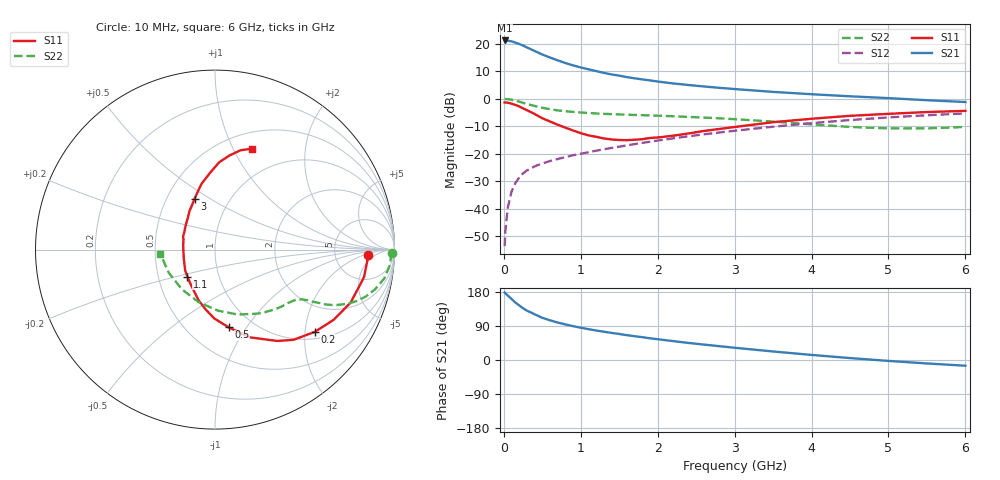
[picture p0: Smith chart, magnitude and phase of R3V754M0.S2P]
! SIEMENS Small Signal Semiconductors
! BFR181
! Si NPN RF Bipolar Junction Transistor in SOT23
! VCE = 0.75 V  IC = 4 mA
! Common Emitter S-Parameters:  May  1996
# GHz  S  MA  R  50
!  f  S11  S21  S12  S22
! GHz  MAG  ANG  MAG  ANG  MAG  ANG  MAG  ANG
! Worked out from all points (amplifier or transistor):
!   36 points, 10 MHz to 6 GHz, reference 50 ohm
!   highest |S21| = 21.1 dB at 10 MHz (marker M1)
!   |S21| within 3 dB of that: start of sweep to 336.7 MHz
!   unconditionally stable (mu >= 1): 993.2 MHz to 3.41 GHz
!   at 250 MHz: K = 0.39, MSG = 23.2 dB, |S12| = -27.1 dB
!   at 1.4 GHz: K = 1.10, MAG = 11.4 dB, |S12| = -17.9 dB
!   at 6 GHz: K = 0.91, MSG = 2.1 dB, |S12| = -5.4 dB
!   S11 on the Smith chart (normalised r, x): 10 MHz: 12, -3; 200 MHz: 1.18, -2.25; 500 MHz: 0.78, -0.83; 1.1 GHz: 0.70, -0.22; 3 GHz: 0.69, +0.43; 6 GHz: 0.68, +1.19
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0.01  0.8518 -2.1  11.36 178.3  0.0021 93.1  0.9873 -1.1
0.02  0.8504 -4.5  11.24 176.0  0.004 89.8  0.9813 -2.1
0.05  0.8443 -10.5  11.2 170.4  0.0103 83.8  0.9789 -5.0
0.1  0.8114 -21.3  10.97 161.1  0.0205 78.6  0.9564 -9.7
0.15  0.7683 -30.6  10.36 151.7  0.0293 73.1  0.9193 -13.9
0.2  0.7204 -39.5  9.813 144.0  0.0371 69.6  0.881 -17.2
0.25  0.6667 -48.9  9.179 136.4  0.0441 65.9  0.839 -20.0
0.3  0.6163 -55.7  8.496 130.3  0.0497 63.9  0.7993 -22.2
0.4  0.5262 -68.3  7.323 120.7  0.059 60.3  0.736 -24.9
0.5  0.4402 -79.9  6.315 111.4  0.0665 58.6  0.6831 -26.5
0.6  0.3841 -90.6  5.567 104.7  0.0737 57.4  0.6416 -27.4
0.7  0.3357 -99.2  4.949 98.9  0.0801 57.5  0.6122 -28.2
0.9  0.2639 -115.4  4.011 89.3  0.0938 57.5  0.5748 -29.2
1.1  0.2153 -135.6  3.405 81.4  0.1065 58.3  0.5484 -30.5
1.3  0.1894 -153.8  2.932 74.6  0.1206 58.8  0.5299 -32.0
1.6  0.1763 -179.1  2.454 65.5  0.1419 59.1  0.5112 -34.9
2.2  0.2123 140.3  1.886 49.9  0.1901 57.8  0.4784 -43.0
3  0.3056 111.9  1.492 32.3  0.2611 53.2  0.4232 -57.6
3.5  0.3735 101.7  1.325 22.5  0.3092 49.1  0.3831 -70.7
4.5  0.4875 87.2  1.102 5.1  0.4083 38.1  0.3062 -107.5
5.5  0.5706 75.7  0.935 -9.1  0.4994 25.0  0.2885 -153.8
6  0.5994 69.9  0.868 -15.1  0.5386 18.0  0.3058 -175.9
